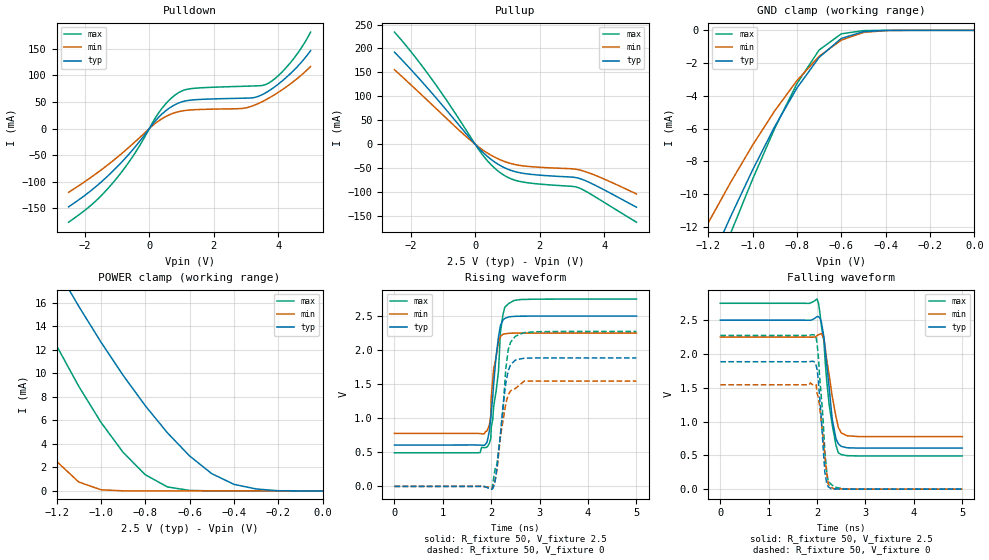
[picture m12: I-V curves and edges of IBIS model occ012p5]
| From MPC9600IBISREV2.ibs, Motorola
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|   Output Buffer at 2.5V application
[Model]   occ012p5
Model_type   Output
Enable   Active-Low
Polarity   Non-Inverting
Vref=1.25
Cref=1pf
Rref=50
| Variable   typ   min   max
C_comp   5p   5p   5p
[Temperature Range]   27.00   100.00   -45.00
[Voltage Range]   2.50V   2.25V   2.75V
[Pulldown Reference]   0.000V   0.000V   0.000V
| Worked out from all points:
|   slope of the pulldown table from 0 to 0.375 V, typ, clamps not added: 14.3 ohm
|   slope of the pullup table from 0 to 0.375 V, typ, clamps not added: 14.9 ohm
|   GND clamp passes 1 mA (typ) near -0.64 V on its own axis
|   POWER clamp passes 1 mA (typ) near -0.45 V on its own axis
|   rising waveform, R_fixture 50, V_fixture 2.5: 20-80 % time 149ps typ, 121ps min, 176ps max; typ from 0.607 V to 2.5 V
|   falling waveform, R_fixture 50, V_fixture 2.5: 20-80 % time 168ps typ, 198ps min, 199ps max; typ from 2.5 V to 0.607 V
|   rising waveform, R_fixture 50, V_fixture 0: 20-80 % time 166ps typ, 179ps min, 176ps max; typ from 0 V to 1.89 V
|   falling waveform, R_fixture 50, V_fixture 0: 20-80 % time 111ps typ, 138ps min, 135ps max; typ from 1.89 V to 0 V
[Pulldown]
|Voltage   I(typ)   I(min)   I(max)
-2.5V     -146.9mA   -119.7mA   -175.9mA
-1.7V     -111.3mA   -86.99mA   -138.4mA
-1.1V     -78.22mA   -59.23mA   -99.89mA
-500mV    -38.9mA    -28.07mA   -51.33mA
300mV     21.87mA    14.82mA    30.33mA
800mV     44.93mA    29.89mA    63.01mA
1.3V      53.5mA     35.02mA    74.99mA
2.9V      56.98mA    37.9mA     79.37mA
3.6V      66.87mA    53.67mA    82.45mA
4.3V      98.98mA    80.62mA    118.4mA
4.7V      123.6mA    99.72mA    150.3mA
5V        146.3mA    116.6mA    181.2mA
[Pullup]
|Voltage  I(typ)   I(min)   I(max)
-2.5V     192.4mA    155.7mA    234.3mA
-2V       156.8mA    124.7mA    194.3mA
-1.4V     111.5mA    86.67mA    141.2mA
-800mV    64.07mA    48.35mA    83.31mA
-200mV    15.7mA     11.4mA     21.18mA
300mV     -20.78mA   -15.02mA   -28.22mA
700mV     -41.45mA   -30.26mA   -55.56mA
1V        -51.95mA   -38.25mA   -68.89mA
1.4V      -59.85mA   -44.55mA   -78.11mA
3.2V      -70.97mA   -53.28mA   -90.82mA
3.8V      -88.51mA   -67.15mA   -113.3mA
5V        -131.7mA   -104.1mA   -163mA
[GND_clamp]
| voltage   I(typ)   I(min)   I(max)
-2.5V     -57.88mA   -49.35mA   -63.49mA
-1.3V     -17.56mA   -14.32mA   -19.46mA
-1.2V     -14.43mA   -11.76mA   -15.9mA
-1.1V     -11.4mA    -9.311mA   -12.43mA
-1V       -8.531mA   -7.015mA   -9.093mA
-900mV    -5.871mA   -4.914mA   -5.985mA
-800mV    -3.524mA   -3.07mA    -3.255mA
-700mV    -1.653mA   -1.587mA   -1.202mA
-600mV    -494uA     -597.7uA   -213.7uA
-500mV    -78.44uA   -130.1uA   -18.2uA
-400mV    -7.209uA   -15.25uA   -728.5nA
1.08fV    -14.8pA    -440.1pA   -2.753pA
[POWER_clamp]
| voltage   I(typ)  I(min)  I(max)
-2.5V     70.85mA    65.33mA    74.29mA
-1.6V     33.33mA    17.01mA    29.01mA
-1.4V     25.87mA    8.67mA     20.22mA
-1.3V     22.33mA    5.244mA    16.15mA
-1.2V     18.94mA    2.521mA    12.36mA
-1.1V     15.71mA    759.7uA    8.904mA
-900mV    9.839mA    6.152uA    3.283mA
-800mV    7.251mA    218.1nA    1.379mA
-700mV    4.941mA    5.214nA    339.4uA
-500mV    1.468mA    4.905pA    3.714uA
-400mV    559.2uA    3.124pA    227.2nA
0V        87.33nA    2.293pA    34.03pA
[Ramp]
dV/dt_r   1.13/162.9p   0.865/274.63p   1.366/109.1p
dV/dt_f   1.13/114p   0.865/169.4p   1.366/73p
R_load = 50
[Rising Waveform]
R_fixture = 50
V_fixture = 2.5
V_fixture_min = 2.25
V_fixture_max = 2.75
|Time (ns) Voltage(typ)  Voltage(min)  Voltage(max)
0s        607.4mV    777.6mV    493mV
1.93ns    702.3mV    845.2mV    593.6mV
1.99ns    997.1mV    1.041V     704.2mV
2ns       1.098V     1.313V     864.5mV
2.05ns    1.507V     1.725V     1.174V
2.15ns    2.197V     2.122V     1.693V
2.19ns    2.364V     2.202V     2.265V
2.28ns    2.466V     2.24V      2.631V
2.36ns    2.488V     2.247V     2.685V
5ns       2.5V       2.25V      2.75V
[Falling Waveform]
R_fixture = 50
V_fixture = 2.5
V_fixture_min = 2.25
V_fixture_max = 2.75
|Time (ns) Voltage(typ)  Voltage(min)  Voltage(max)
0s        2.5V       2.25V      2.75V
2ns       2.553V     2.272V     2.812V
2.09ns    2.466V     2.302V     2.411V
2.14ns    2.255V     2.229V     2.194V
2.2ns     1.841V     1.91V      1.599V
2.25ns    1.503V     1.688V     1.246V
2.31ns    1.048V     1.385V     962.2mV
2.44ns    670.2mV    911.3mV    537.1mV
2.62ns    612mV      789.7mV    495.5mV
5ns       607.3mV    777.9mV    490.7mV
[Rising Waveform]
R_fixture = 50
V_fixture = 0
V_fixture_min = 0
V_fixture_max = 0
|Time (ns) Voltage(typ)  Voltage(min)  Voltage(max)
0s        141.9pV    5.687nV    20.53pV
2.02ns    -41.08mV   -33.99mV   -24.45mV
2.08ns    75.64mV    86.93mV    257mV
2.15ns    499mV      453.6mV    507.2mV
2.24ns    1.157V     950.7mV    1.103V
2.3ns     1.511V     1.214V     1.723V
2.35ns    1.694V     1.345V     2.004V
2.5ns     1.855V     1.438V     2.204V
2.68ns    1.882V     1.545V     2.258V
5ns       1.885V     1.545V     2.274V
[Falling Waveform]
R_fixture = 50
V_fixture = 0
V_fixture_min = 0
V_fixture_max = 0
|Time (ns) Voltage(typ)  Voltage(min)  Voltage(max)
0s        1.885V     1.544V     2.274V
1.96ns    1.87V      1.552V     2.274V
1.98ns    1.829V     1.547V     2.247V
2ns       1.771V     1.415V     2.153V
2.03ns    1.583V     1.351V     1.929V
2.12ns    674.6mV    792.9mV    1.078V
2.16ns    252.5mV    489.5mV    560.4mV
2.23ns    35.59mV    77.75mV    120.3mV
2.35ns    3.805mV    6.638mV    37.41mV
5ns       1.952uV    -556.1nV   -109.5uV
